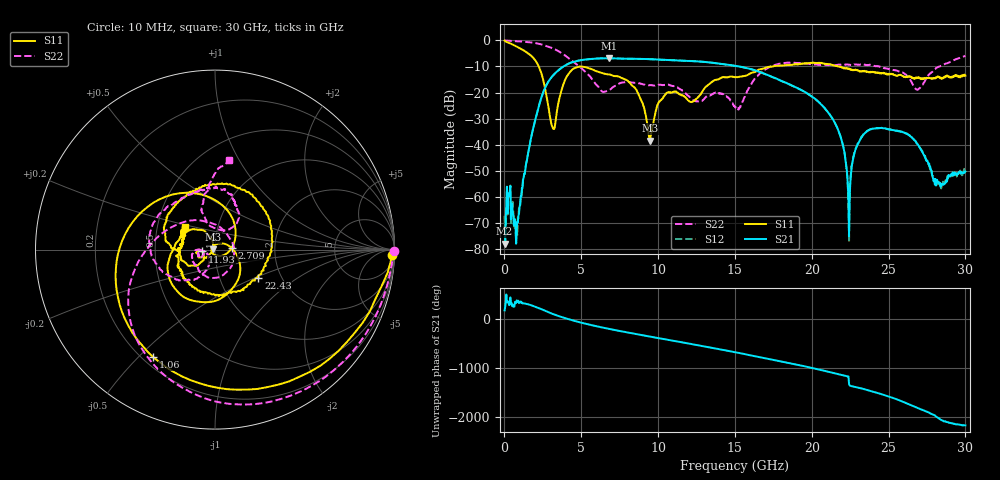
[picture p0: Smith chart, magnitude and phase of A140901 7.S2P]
!  2-Port S-parameters saved by WinCal
! VAR MeasName=S-Parameters (CALIBRATED_DATA) read from VNA (N5244A)
! VAR MeasDate=11/3/2014 9:27:06 AM
! VAR NAME=A140901 7
! VAR FILENAME=A140901 7.S2P
! VAR DATE=11/3/2014 9:27:06 AM
! VAR PHYS_PORTS=1,2
# Hz S RI R 50
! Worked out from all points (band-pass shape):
!   801 points, 10 MHz to 30 GHz, reference 50 ohm
!   highest |S21| = -6.86 dB at 6.795 GHz (marker M1); lowest = -77.9 dB at 10 MHz (marker M2)
!   |S21| within 3 dB of the highest: 3.88 GHz to 15.11 GHz (11.23 GHz wide, 118 % of centre)
!   lowest |S11| = -38.4 dB at 9.457 GHz (marker M3), VSWR 1.02, Z = 48.8 + j0.112 ohm
!   |S11| at or under -10 dB: 2.23 GHz to 4.915 GHz (2.685 GHz wide, 75.2 % of centre); 4.961 GHz to 17.46 GHz (12.5 GHz wide, 111 % of centre); 21.75 GHz to end of sweep
!   |S22| runs from -26.6 to 0.0 dB; largest |S21 - S12| = 0.0041
!   S11 on the Smith chart (normalised r, x): 10 MHz: 20, -56; 1.06 GHz: 0.24, -0.55; 2.709 GHz: 1.21, +0.02; 11.93 GHz: 0.87, -0.02; 22.43 GHz: 1.53, -0.52; 30 GHz: 0.69, +0.18
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1e7  0.9881 -0.0311  -0.000125 1.8e-05  0.00021 -0.000381  0.996 -0.00802
2.34925e8  0.7803 -0.4612  0.000986 -0.000167  0.00117 -2.66e-06  0.9701 -0.1547
7.5975e8  0.0127 -0.7694  0.000101 -7.74e-05  0.000128 2.15e-05  0.8495 -0.4534
1.05965e9  -0.3433 -0.6003  0.00103 -0.000157  0.000993 -0.000195  0.7394 -0.5983
2.034325e9  -0.2737 0.2954  -0.0147 -0.0293  -0.0147 -0.0293  0.2046 -0.862
2.7091e9  0.0942 0.00966  -0.1221 0.0594  -0.1218 0.059  -0.2007 -0.7579
3.196438e9  -0.0188 0.00686  -0.00808 0.2185  -0.00838 0.2176  -0.4007 -0.5631
3.983675e9  0.1405 -0.1204  0.3297 0.0578  0.3295 0.0586  -0.4706 -0.1793
5.033325e9  -0.1998 -0.2434  0.0585 -0.4159  0.0581 -0.4163  -0.2681 0.1095
6.795238e9  -0.2196 0.031  -0.4104 0.194  -0.4104 0.1944  0.1065 -0.0262
8.519662e9  -0.0596 0.1037  0.2757 0.3475  0.2756 0.3476  -0.072 -0.1357
9.45685e9  -0.012 0.00115  0.4361 -0.0177  0.4352 -0.0174  -0.0995 -0.0962
1.001916e10  -0.0468 -0.0425  0.356 -0.2408  0.3554 -0.2403  -0.1136 -0.084
1.193102e10  -0.0708 -0.0104  -0.3159 -0.2549  -0.3157 -0.2544  -0.0873 0.000343
1.5005e10  -0.1972 -0.0138  0.2526 0.2052  0.2536 0.2025  -0.0502 -0.0145
2.002832e10  0.0635 0.3681  0.0179 0.0809  0.0177 0.0813  -0.2345 0.2522
2.171526e10  0.3168 0.0181  0.013 -0.014  0.0132 -0.0139  -0.119 0.3199
2.242752e10  0.2422 -0.1567  -5.91e-05 0.000163  -2.64e-05 0.00013  -0.0734 0.3337
2.325225e10  0.0611 -0.2501  0.0132 0.00446  0.0135 0.00466  0.00472 0.3473
2.501416e10  -0.1913 -0.1099  -0.0159 -0.0117  -0.016 -0.0115  0.1122 0.2617
2.831306e10  -0.1878 0.0667  -0.000893 0.0015  -0.001 0.00165  -0.0576 0.311
3e10  -0.1688 0.1264  0.003 -0.00067  0.00301 -0.000735  0.0768 0.4993
